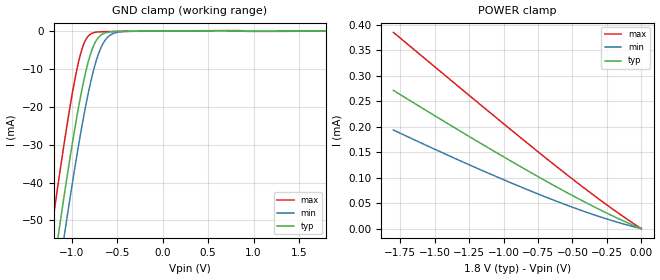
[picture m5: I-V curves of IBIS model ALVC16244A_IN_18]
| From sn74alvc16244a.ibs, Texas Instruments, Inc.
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[Model]   ALVC16244A_IN_18
Model_type  Input
Vinl=0.5775
Vinh=1.2675
| variable   typ   min   max
C_comp   0.92pF   0.66pF   1.10pF
[Temperature Range]   40   100   -40
| Ambient temperature   25   85   -40
[Voltage range]   1.8   1.65   1.95
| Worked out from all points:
|   GND clamp passes 1 mA (typ) near -0.67 V on its own axis
[GND Clamp]
| ALVC16244A_IN_18
|   Voltage   I(typ)   I(min)   I(max)
-1.8V     -169.8mA   -179.9mA   -157.2mA
-1.22V    -66.13mA   -76.92mA   -52.28mA
-1.14V    -52.75mA   -63.56mA   -38.84mA
-1.075V   -42.24mA   -53mA      -28.44mA
-935mV    -21.51mA   -31.67mA   -9.29mA
-860mV    -12.31mA   -21.51mA   -3.028mA
-785mV    -5.514mA   -12.84mA   -700.9uA
-725mV    -2.335mA   -7.439mA   -286.7uA
-660mV    -801.2uA   -3.501mA   -184uA
-590mV    -272.2uA   -1.321mA   -150.3uA
-495mV    -105.2uA   -324uA     -122.8uA
1.8V      1.112nA    10.77uA    -24.83uA
[POWER Clamp]
| ALVC16244A_IN_18
|   Voltage   I(typ)   I(min)   I(max)
-1.8V     271.4uA    193.7uA    385.3uA
-1.215V   175.3uA    121.3uA    253.8uA
-715mV    96.81uA    64.34uA    143.3uA
-325mV    40.43uA    25.51uA    61.41uA
-16.28fV  1.112nA    59.61nA    5.254pA
